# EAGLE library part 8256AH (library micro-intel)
MICROCOMPUTER/PERIPHERAL DEVICE
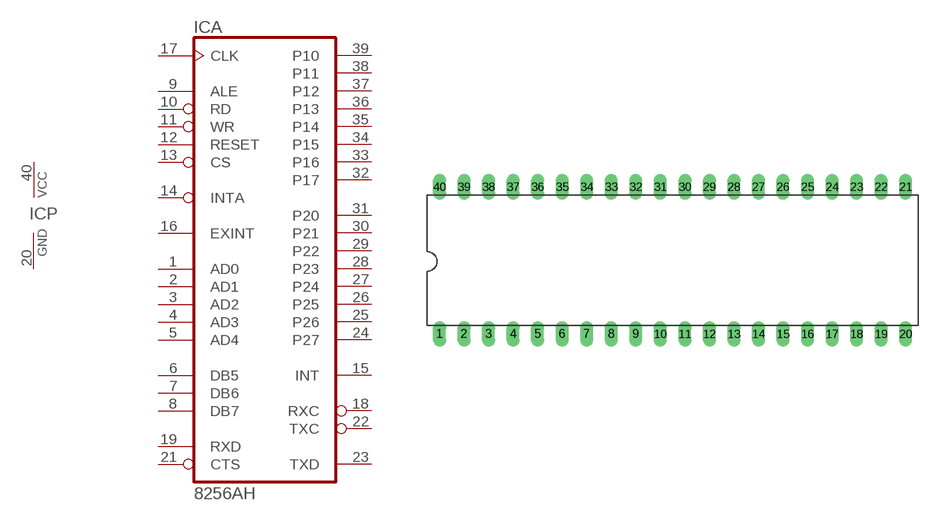
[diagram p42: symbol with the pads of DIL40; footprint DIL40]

Designator prefix IC; gates A=8256AH P=PWRN

## 8256AH (OC_FARNELL: unknown; OC_NEWARK: unknown)  [DIL40]
1  A:AD0
2  A:AD1
3  A:AD2
4  A:AD3
5  A:AD4
6  A:DB5
7  A:DB6
8  A:DB7
9  A:ALE  in
10  A:RD  in
11  A:WR  in
12  A:RESET  in
13  A:CS  in
14  A:INTA  in
15  A:INT  out
16  A:EXINT  in
17  A:CLK  in
18  A:RXC
19  A:RXD  in
20  P:GND  pwr
21  A:CTS  in
22  A:TXC
23  A:TXD  out
24  A:P27
25  A:P26
26  A:P25
27  A:P24
28  A:P23
29  A:P22
30  A:P21
31  A:P20
32  A:P17
33  A:P16
34  A:P15
35  A:P14
36  A:P13
37  A:P12
38  A:P11
39  A:P10
40  P:VCC  pwr

## Footprint DIL40 (pad centres in mm)
Dual In Line Package
drill 0.813 long: 1 -24.13,-7.62; 2 -21.59,-7.62; 3 -19.05,-7.62; 4 -16.51,-7.62; 5 -13.97,-7.62; 6 -11.43,-7.62; 7 -8.89,-7.62; 8 -6.35,-7.62; 9 -3.81,-7.62; 10 -1.27,-7.62; 11 1.27,-7.62; 12 3.81,-7.62; 13 6.35,-7.62; 14 8.89,-7.62; 15 11.43,-7.62; 16 13.97,-7.62; 17 16.51,-7.62; 18 19.05,-7.62; 19 21.59,-7.62; 20 24.13,-7.62; 21 24.13,7.62; 22 21.59,7.62; 23 19.05,7.62; 24 16.51,7.62; 25 13.97,7.62; 26 11.43,7.62; 27 8.89,7.62; 28 6.35,7.62; 29 3.81,7.62; 30 1.27,7.62; 31 -1.27,7.62; 32 -3.81,7.62; 33 -6.35,7.62; 34 -8.89,7.62; 35 -11.43,7.62; 36 -13.97,7.62; 37 -16.51,7.62; 38 -19.05,7.62; 39 -21.59,7.62; 40 -24.13,7.62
